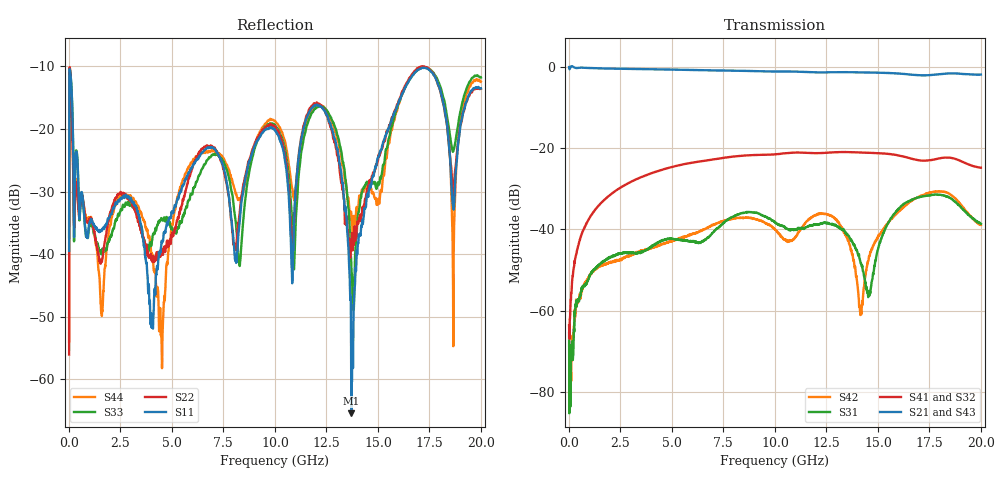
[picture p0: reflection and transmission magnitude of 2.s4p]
!Keysight Technologies,N5225A,MY51451420,A.10.40.12
!Date: Tuesday, October 13, 2015 09:44:53
!Correction: S11(Full 4 Port(1,2,3,4))
!S12(Full 4 Port(1,2,3,4))
!S13(Full 4 Port(1,2,3,4))
!S14(Full 4 Port(1,2,3,4))
!S21(Full 4 Port(1,2,3,4))
!S22(Full 4 Port(1,2,3,4))
!S23(Full 4 Port(1,2,3,4))
!S24(Full 4 Port(1,2,3,4))
!S31(Full 4 Port(1,2,3,4))
!S32(Full 4 Port(1,2,3,4))
!S33(Full 4 Port(1,2,3,4))
!S34(Full 4 Port(1,2,3,4))
!S41(Full 4 Port(1,2,3,4))
!S42(Full 4 Port(1,2,3,4))
!S43(Full 4 Port(1,2,3,4))
!S44(Full 4 Port(1,2,3,4))
!S4P File: Measurements: <S11,S12,S13,S14>,
!<S21,S22,S23,S24>,
!<S31,S32,S33,S34>,
!<S41,S42,S43,S44>:
# Hz S  dB  R 50
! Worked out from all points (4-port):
!   2000 points, 10 MHz to 20 GHz, reference 50 ohm
!   strongest paths, dB at 10 MHz, 5.01 GHz, 10.01 GHz, 15.01 GHz, 20 GHz:
!     S21: 0.0, -0.7, -1.1, -1.4, -1.9
!     S43: -0.1, -0.7, -1.1, -1.4, -2.0
!     S41: -63.6, -24.6, -21.5, -21.2, -24.8
!     S32: -67.7, -24.6, -21.5, -21.2, -24.9
!     S31: -65.4, -42.3, -38.3, -44.8, -38.6
!     S42: -63.7, -42.8, -40.0, -41.8, -38.9
!   lowest |S11| = -65.4 dB at 13.71 GHz (marker M1), VSWR 1.00, Z = 50.1 + j0.0182 ohm
!   |S11| at or under -10 dB: start of sweep to end of sweep
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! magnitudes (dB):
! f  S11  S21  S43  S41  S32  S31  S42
! 10 MHz  -39.5  0.0  -0.1  -63.6  -67.7  -65.4  -63.7
! 2.19 GHz  -32.7  -0.4  -0.4  -30.8  -30.8  -46.4  -47.8
! 4.47 GHz  -38.9  -0.6  -0.6  -25.4  -25.4  -42.9  -43.7
! 12.22 GHz  -16.5  -1.4  -1.4  -21.2  -21.2  -38.6  -36.1
! 13.71 GHz  -65.4  -1.3  -1.3  -21.0  -21.0  -42.5  -45.3
! 16.37 GHz  -13.1  -1.8  -1.8  -22.2  -22.2  -33.3  -33.9
! 20 GHz  -13.5  -1.9  -2.0  -24.8  -24.9  -38.6  -38.9
